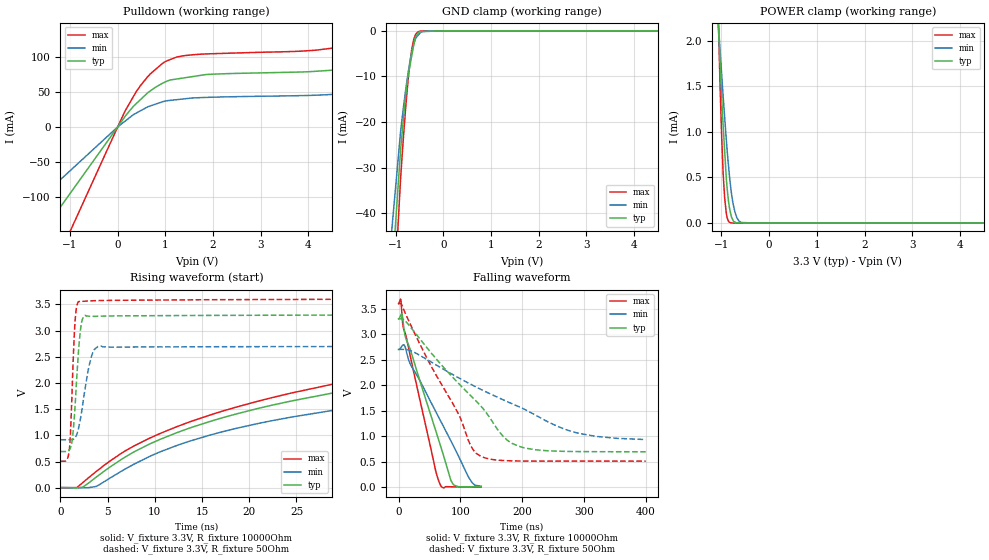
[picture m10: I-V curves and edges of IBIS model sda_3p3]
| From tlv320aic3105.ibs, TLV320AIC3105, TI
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|   sda_3p3 Model
[Model]   sda_3p3
Model_type   I/O_open_drain
Polarity   Inverting
Vinl = 0.99
Vinh = 2.31
Vmeas = 1.65
Vref = 3.3
Cref = 2pF
Rref = 10000
|   typ   min   max
|   (nom PVT)   (fast PVT)   (slow PVT)
C_comp   1.219e-12   1.219e-12   1.225e-12
| Where nom  PVT is Nominal Process, 3.3V, 27C
|   Fast PVT is Strong Process,  3.6V, -40C
|   Slow PVT is Weak Process,   2.7V, 105C
[Model Spec]
|Subparameter   typ   min   max
Vinh   2.31   1.89   2.52
Vinl   0.99   0.81   1.08
[Voltage Range]   3.3   2.7   3.6
|Ambient Temperature   25   85   -40
|Junction Temperature
[Temperature Range]   27   105   -40
[Pullup Reference]   3.3   2.7   3.6
[Pulldown Reference]   0   0   0
[Power Clamp Reference]   3.3   2.7   3.6
[GND Clamp Reference]   0   0   0
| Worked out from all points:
|   slope of the pulldown table from 0 to 0.495 V, typ, clamps not added: 12.3 ohm
|   GND clamp passes 1 mA (typ) near -0.56 V on its own axis
|   POWER clamp passes 1 mA (typ) near -0.96 V on its own axis
|   falling waveform, V_fixture 3.3V, R_fixture 10000Ohm: 20-80 % time 51.1ns typ, 68ns min, 39.2ns max; typ from 3.3 V to 0.004 V
|   rising waveform, V_fixture 3.3V, R_fixture 10000Ohm: 20-80 % time 59.5ns typ, 61.9ns min, 57.7ns max; typ from 0.003 V to 3.3 V
|   falling waveform, V_fixture 3.3V, R_fixture 50Ohm: 20-80 % time 113ns typ, 173ns min, 79.5ns max; typ from 3.3 V to 0.692 V
|   rising waveform, V_fixture 3.3V, R_fixture 50Ohm: 20-80 % time 579ps typ, 983ps min, 402ps max; typ from 0.692 V to 3.3 V
[Pulldown]
|   Voltage   I(typ)   I(min)   I(max)
-3.3V     -315.2mA   -207.5mA   -494.8mA
-2.7mV    -257.9uA   -169.8uA   -404.9uA
154.8mV   15.04mA    8.288mA    22.78mA
478.8mV   39.21mA    23.18mA    59.26mA
684mV     51.6mA     30.06mA    75.97mA
1.008V    64.73mA    37.14mA    93.95mA
1.591V    72.32mA    41.52mA    103.5mA
4.162V    79.74mA    45.48mA    110mA
5.148V    89.77mA    53.24mA    126.5mA
5.67V     105.2mA    58.58mA    150.6mA
6.379V    147.9mA    65.83mA    213.5mA
6.6V      165.5mA    68.09mA    242.4mA
[GND Clamp]
|   Voltage   I(typ)   I(min)   I(max)
-3.3V     -1.085A    -925.9mA   -1.224A
-1.476V   -114.9mA   -89.64mA   -144.4mA
-897.6mV  -26.09mA   -22.13mA   -32.41mA
-842.4mV  -19.83mA   -17.17mA   -23.94mA
-772.2mV  -12.51mA   -11.53mA   -14.59mA
-745.8mV  -10.15mA   -9.639mA   -11.43mA
-702mV    -7.665mA   -6.818mA   -7.047mA
-622.8mV  -3.177mA   -2.974mA   -1.957mA
-590.7mV  -1.359mA   -1.919mA   -1.016mA
-532.8mV  -597.9uA   -1.011mA   -208.3uA
-286.2mV  -107.2uA   -2.585uA   -6.129uA
6.6V      0A         0A         0A
[POWER Clamp]
|   Voltage   I(typ)   I(min)   I(max)
-3.3V     32.15mA    22.38mA    56.05mA
-1.076V   2.305mA    2.283mA    2.475mA
-1.03V    1.766mA    1.906mA    1.532mA
-993.6mV  1.375mA    1.621mA    934uA
-964.8mV  1.081mA    1.4mA      561.5uA
-932.4mV  796.9uA    1.166mA    280.4uA
-881.1mV  387.7uA    807.4uA    64.82uA
-820.8mV  138.7uA    461.6uA    4.877uA
-766.8mV  41.34uA    246.3uA    409.3nA
-718.2mV  11.1uA     124.3uA    128.1nA
-583.2mV  2.076uA    6.133uA    0A
6.6V      0A         0A         0A
[Ramp]
R_load = 10000
|   typ   min   max
dV/dt_r   1.97786/5.93751e-08   1.6169/6.18159e-08   2.15849/5.7654e-08
dV/dt_f   1.97812/5.11085e-08   1.61742/6.82407e-08   2.15865/3.92319e-08
[Falling Waveform]
V_fixture = 3.3V
V_fixture_min = 2.7V
V_fixture_max = 3.6V
R_fixture = 10000Ohm
|   Time   V(typ)   V(min)   V(max)
0s        3.3V       2.7V       3.6V
3.625ns   3.372V     2.734V     3.687V
5.775ns   3.387V     2.768V     3.336V
11.37ns   2.937V     2.726V     2.996V
19.05ns   2.696V     2.413V     2.569V
60.5ns    1.096V     1.475V     297.9mV
68.4ns    791.6mV    1.29V      23.54mV
88.85ns   48.7mV     806.5mV    3.235mV
119ns     4.568mV    86.93mV    2.39mV
133.7ns   3.776mV    14.85mV    2.307mV
[Rising Waveform]
V_fixture = 3.3V
V_fixture_min = 2.7V
V_fixture_max = 3.6V
R_fixture = 10000Ohm
|   Time   V(typ)   V(min)   V(max)
0s        3.134mV    4.295mV    2.25mV
1.725ns   -1.31mV    2.014mV    2.385mV
3.8ns     205.3mV    25.96mV    312.5mV
7.8ns     686mV      451.3mV    798.8mV
12.98ns   1.094V     847.1mV    1.21V
30ns      1.848V     1.509V     2.02V
57.55ns   2.493V     2.008V     2.752V
91.35ns   2.911V     2.337V     3.213V
175.5ns   3.239V     2.629V     3.546V
400ns     3.3V       2.699V     3.6V
[Falling Waveform]
V_fixture = 3.3V
V_fixture_min = 2.7V
V_fixture_max = 3.6V
R_fixture = 50Ohm
|   Time   V(typ)   V(min)   V(max)
0s        3.3V       2.7V       3.6V
5.125ns   3.302V     2.702V     3.582V
12.3ns    3.243V     2.698V     3.375V
95ns      2.061V     2.159V     1.481V
117.8ns   1.781V     2.011V     791.8mV
130.8ns   1.621V     1.932V     620.3mV
167.9ns   1.012V     1.719V     520.8mV
201.7ns   774.3mV    1.538V     509.6mV
287.6ns   696mV      1.066V     507.4mV
400ns     692mV      931.7mV    507.4mV
[Rising Waveform]
V_fixture = 3.3V
V_fixture_min = 2.7V
V_fixture_max = 3.6V
R_fixture = 50Ohm
|   Time   V(typ)   V(min)   V(max)
0s        691.9mV    917mV      507.4mV
950ps     723.1mV    917mV      746.9mV
1.25ns    918.5mV    918.2mV    1.928V
1.55ns    1.561V     955.9mV    3.175V
1.725ns   2.097V     1.016V     3.465V
2.075ns   2.935V     1.277V     3.56V
2.475ns   3.268V     1.74V      3.559V
3.225ns   3.27V      2.469V     3.567V
4.2ns     3.274V     2.708V     3.573V
66.22ns   3.3V       2.699V     3.6V
